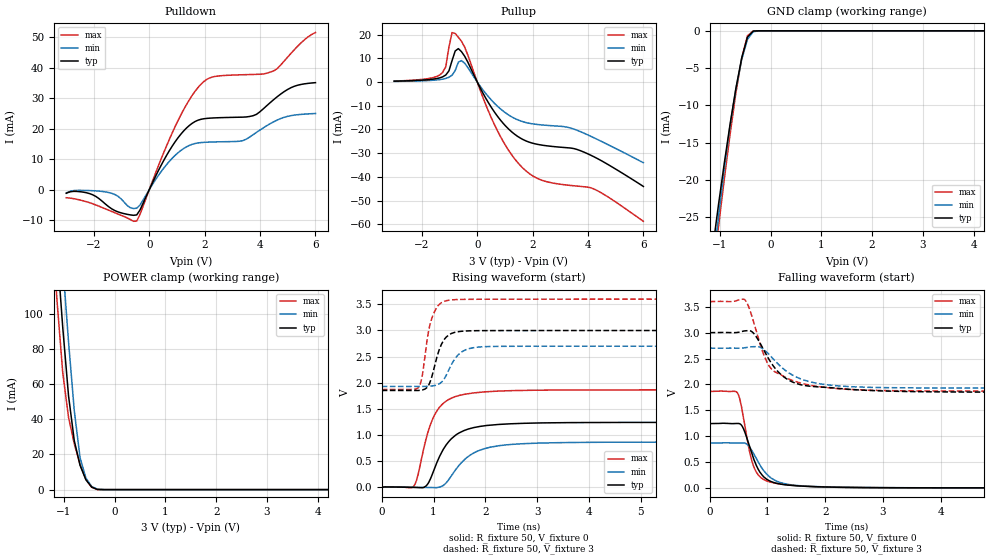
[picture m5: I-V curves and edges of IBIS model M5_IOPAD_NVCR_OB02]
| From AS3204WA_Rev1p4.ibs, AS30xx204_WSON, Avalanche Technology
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[Model] M5_IOPAD_NVCR_OB02
Model_type I/O
Enable   Active-High
Vinl  =  0.9
Vinh  =  2.1
Vmeas =  1.5
Cref  =  30e-12
| Capacitance  typ   min   max
C_comp   3.872127e-12   3.590660e-12   4.176448e-12
| Variables   typ   min   max
[GND Clamp Reference]   0   0   0
[POWER Clamp Reference]   3   2.7   3.6
[Pulldown Reference]   0   0   0
[Pullup Reference]   3   2.7   3.6
[Temperature Range]   25   105   -40
[Voltage Range]   3   2.7   3.6
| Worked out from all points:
|   slope of the pulldown table from 0 to 0.45 V, typ, clamps not added: 53.8 ohm
|   slope of the pullup table from 0 to 0.45 V, typ, clamps not added: 46.8 ohm
|   GND clamp passes 1 mA (typ) near -0.46 V on its own axis
|   POWER clamp passes 1 mA (typ) near -0.42 V on its own axis
|   falling waveform, R_fixture 50, V_fixture 0: 20-80 % time 272ps typ, 341ps min, 213ps max; typ from 1.24 V to 0 V
|   falling waveform, R_fixture 50, V_fixture 3: 20-80 % time 489ps typ, 583ps min, 431ps max; typ from 3 V to 1.85 V
|   rising waveform, R_fixture 50, V_fixture 0: 20-80 % time 445ps typ, 538ps min, 354ps max; typ from 0 V to 1.24 V
|   rising waveform, R_fixture 50, V_fixture 3: 20-80 % time 215ps typ, 278ps min, 179ps max; typ from 1.85 V to 3 V
[GND Clamp]
| Voltage   I(typ)   I(min)   I(max)
-3V       -145.9mA   -151.9mA   -144.2mA
-1.138V   -29.07mA   -31.55mA   -32.68mA
-1.024V   -23.24mA   -24.83mA   -26.15mA
-910.3mV  -17.69mA   -18.46mA   -19.83mA
-796.6mV  -12.47mA   -12.67mA   -13.82mA
-682.8mV  -7.718mA   -7.754mA   -8.316mA
-569mV    -3.663mA   -3.867mA   -3.675mA
-455.2mV  -839.2uA   -1.152mA   -666.1uA
-341.4mV  -35.63uA   -111.1uA   -11.17uA
-113.8mV  -8.642nA   -188.3nA   -1.888nA
6V        0A         0A         0A
[POWER Clamp]
| Voltage   I(typ)   I(min)   I(max)
-3V       949.8mA    984.2mA    923.5mA
-1.252V   183.6mA    221.4mA    154mA
-1.138V   136.7mA    174.2mA    107.6mA
-1.024V   92.09mA    128.1mA    66.35mA
-910.3mV  53.33mA    83.97mA    41.06mA
-796.6mV  27.72mA    44.75mA    25.94mA
-682.8mV  13.75mA    18.06mA    14.29mA
-569mV    5.664mA    6.605mA    5.738mA
-455.2mV  1.446mA    1.789mA    1.305mA
-341.4mV  77.09uA    287.6uA    62.73uA
-227.6mV  1.148uA    12.92uA    332nA
6V        0A         0A         0A
[Pulldown]
| Voltage   I(typ)   I(min)   I(max)
-3V       -1.234mA   -1.124mA   -2.704mA
-2.162V   -1.332mA   -343.7uA   -4.325mA
-1.479V   -5.575mA   -964.8uA   -6.759mA
-455.2mV  -8.34mA    -6.122mA   -10.36mA
931mV     15.68mA    11.22mA    20.66mA
1.862V    23.06mA    15.41mA    34.56mA
2.379V    23.54mA    15.64mA    37.15mA
3.372V    23.77mA    16.04mA    37.7mA
3.745V    24.23mA    17.98mA    37.79mA
4.49V     29.51mA    22.25mA    38.97mA
5.234V    33.9mA     24.43mA    45.9mA
6V        35.1mA     24.97mA    51.55mA
[Pullup]
| Voltage   I(typ)   I(min)   I(max)
-3V       346.1uA    258.6uA    405.8uA
-1.366V   1.712mA    1mA        2.902mA
-1.138V   2.946mA    1.502mA    6.431mA
-910.3mV  9.029mA    2.847mA    20.86mA
-796.6mV  13.11mA    4.845mA    20.47mA
-569mV    12.8mA     9.038mA    17.18mA
620.7mV   -12.67mA   -8.969mA   -17.98mA
1.655V    -24.29mA   -16.77mA   -36.41mA
2.379V    -26.71mA   -18.16mA   -41.63mA
3.745V    -29.06mA   -21.03mA   -44.07mA
4.366V    -32.46mA   -24.38mA   -46.01mA
6V        -44.07mA   -34.05mA   -58.77mA
[Ramp]
dV/dt_r   0.745426/0.445098n  0.519332/0.537581n  1.11854/0.354104n
dV/dt_f   0.690854/0.488836n  0.463821/0.583089n  1.0388/0.430793n
R_load = 50
[Falling Waveform]
R_fixture = 50
V_fixture = 0
V_fixture_min = 0
V_fixture_max = 0
| Time   V(typ)   V(min)   V(max)
0s        1.242V     865.6mV    1.864V
484ps     1.245V     866.2mV    1.83V
528.7ps   1.234V     868.1mV    1.686V
581ps     1.155V     869.1mV    1.385V
680.5ps   835.3mV    803.8mV    759.3mV
731.6ps   658.4mV    719.8mV    517.2mV
861.2ps   320.3mV    460.2mV    224.8mV
1.109ns   103.3mV    157.6mV    96mV
1.479ns   41.98mV    49.55mV    43.89mV
21.88ns   454.8nV    595.6nV    9.58uV
[Falling Waveform]
R_fixture = 50
V_fixture = 3
V_fixture_min = 2.7
V_fixture_max = 3.6
| Time   V(typ)   V(min)   V(max)
0s        3V         2.7V       3.6V
602.4ps   3.033V     2.708V     3.641V
664.5ps   3.038V     2.719V     3.533V
768.8ps   2.978V     2.729V     3.179V
937.9ps   2.663V     2.673V     2.571V
1.098ns   2.363V     2.496V     2.267V
1.48ns    2.025V     2.153V     2.058V
2.181ns   1.927V     1.975V     1.92V
4.854ns   1.85V      1.929V     1.869V
21.88ns   1.849V     1.927V     1.869V
[Rising Waveform]
R_fixture = 50
V_fixture = 0
V_fixture_min = 0
V_fixture_max = 0
| Time   V(typ)   V(min)   V(max)
0s        358.1nV    458.8nV    9.504uV
603.6ps   -717.2uV   2.786mV    6.795mV
687.9ps   -5.652mV   1.523mV    190.4mV
864.1ps   34.46mV    -2.841mV   958.5mV
982.8ps   267.3mV    -6.748mV   1.309V
1.105ns   566.1mV    839.3uV    1.52V
1.4ns     978.5mV    300.5mV    1.728V
1.905ns   1.167V     713.4mV    1.82V
3.911ns   1.239V     860.2mV    1.863V
21.88ns   1.242V     865.6mV    1.864V
[Rising Waveform]
R_fixture = 50
V_fixture = 3
V_fixture_min = 2.7
V_fixture_max = 3.6
| Time   V(typ)   V(min)   V(max)
0s        1.849V     1.927V     1.869V
723.2ps   1.854V     1.93V      1.929V
790.5ps   1.864V     1.93V      2.187V
875.7ps   1.911V     1.931V     2.819V
989ps     2.199V     1.942V     3.295V
1.155ns   2.741V     2.013V     3.533V
1.4ns     2.962V     2.441V     3.59V
1.678ns   2.993V     2.651V     3.597V
2.18ns    2.998V     2.696V     3.599V
21.88ns   3V         2.7V       3.6V
